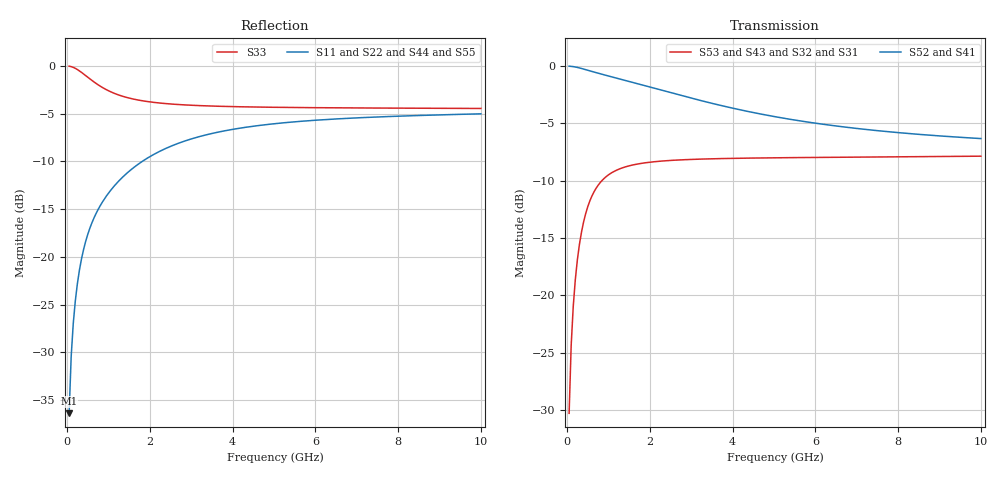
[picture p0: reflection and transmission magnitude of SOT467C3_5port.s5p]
! Created Fri Mar  1 12:52:34 2019
# ghz S ma R 50
! 5 Port Network Data from SP1.SP block
! freq  magS11  angS11  magS12  angS12  magS13  angS13  magS14  angS14
!  magS15  angS15
!  magS21  angS21  magS22  angS22  magS23  angS23
!  magS24  angS24  magS25  angS25
!  magS31  angS31  magS32  angS32
!  magS33  angS33  magS34  angS34  magS35  angS35
!  magS41  angS41
!  magS42  angS42  magS43  angS43  magS44  angS44  magS45  angS45
!  magS51  angS51  magS52  angS52  magS53  angS53  magS54  angS54
!  magS55  angS55
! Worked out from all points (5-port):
!   200 points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, 50 MHz to 10 GHz, reference 50 ohm
!   strongest paths, dB at 50 MHz, 2.55 GHz, 5.05 GHz, 7.55 GHz, 10 GHz:
!     S52: 0.0, -2.4, -4.4, -5.7, -6.3
!     S41: 0.0, -2.4, -4.4, -5.7, -6.3
!     S53: -30.3, -8.2, -8.0, -7.9, -7.9
!     S43: -30.3, -8.2, -8.0, -7.9, -7.9
!     S32: -30.3, -8.2, -8.0, -8.0, -8.0
!     S31: -30.3, -8.2, -8.0, -8.0, -8.0
!   lowest |S11| = -36.4 dB at 50 MHz (marker M1), VSWR 1.03, Z = 49.9 - j1.51 ohm
!   |S11| at or under -10 dB: start of sweep to 1.817 GHz
